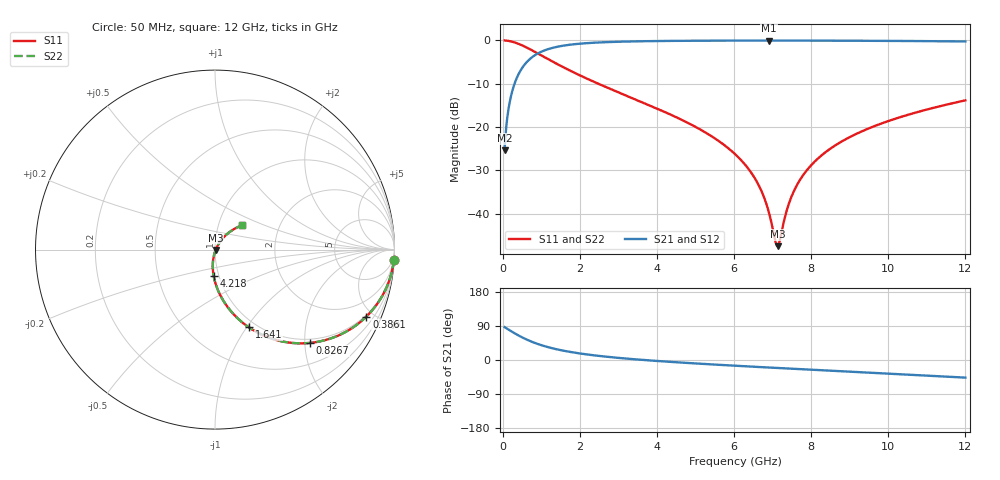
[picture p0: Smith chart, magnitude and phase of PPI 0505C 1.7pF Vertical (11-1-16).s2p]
# GHz S MA R 50
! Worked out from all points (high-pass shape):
!   1601 points, 50 MHz to 12 GHz, reference 50 ohm
!   highest |S21| = -0.04 dB at 6.906 GHz (marker M1); lowest = -25.3 dB at 50 MHz (marker M2)
!   |S21| within 3 dB of the highest: 907.1 MHz to end of sweep
!   lowest |S11| = -47.5 dB at 7.13 GHz (marker M3), VSWR 1.01, Z = 50.4 - j0.142 ohm
!   |S11| at or under -10 dB: 2.477 GHz to end of sweep
!   |S22| runs from -47.5 to 0.0 dB; largest |S21 - S12| = 0
!   S11 on the Smith chart (normalised r, x): 50 MHz: 1, -35; 386.1 MHz: 0.91, -4.55; 826.8 MHz: 0.91, -2.11; 1.641 GHz: 0.92, -1.02; 4.218 GHz: 0.94, -0.29; 12 GHz: 1.30, +0.37
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0.05  0.9985 -3.2  0.05403 86.7  0.05403 86.7  0.9985 -3.2
0.1919063  0.979 -12.3  0.2034 77.7  0.2034 77.7  0.979 -12.3
0.3860938  0.9221 -23.9  0.3862 66.1  0.3862 66.1  0.9221 -23.9
0.5802812  0.8451 -34.0  0.5336 55.9  0.5336 55.9  0.8451 -34.0
0.82675  0.7408 -44.6  0.6704 45.3  0.6704 45.3  0.7408 -44.6
1.207656  0.5974 -56.8  0.8001 33.1  0.8001 33.1  0.5974 -56.8
1.640844  0.4728 -66.4  0.879 23.3  0.879 23.3  0.4728 -66.4
2.044156  0.3866 -73.0  0.9198 16.6  0.9198 16.6  0.3866 -73.0
4.038312  0.1606 -91.7  0.9836 -2.8  0.9836 -2.8  0.1606 -91.7
4.217562  0.1482 -92.8  0.9855 -4.0  0.9855 -4.0  0.1482 -92.8
5.285594  0.08501 -98.4  0.9925 -10.8  0.9925 -10.8  0.08501 -98.4
6.025  0.04866 -100.6  0.9946 -15.1  0.9946 -15.1  0.04866 -100.6
6.56275  0.02456 -98.6  0.9953 -18.0  0.9953 -18.0  0.02456 -98.6
6.756938  0.0163 -94.6  0.9954 -19.1  0.9954 -19.1  0.0163 -94.6
6.906313  0.01024 -86.1  0.9954 -19.9  0.9954 -19.9  0.01024 -86.1
7.063156  0.004985 -53.7  0.9954 -20.7  0.9954 -20.7  0.004985 -53.7
7.130375  0.004205 -19.5  0.9953 -21.1  0.9953 -21.1  0.004205 -19.5
7.51875  0.01683 52.0  0.9951 -23.1  0.9951 -23.1  0.01683 52.0
8.019156  0.03696 57.3  0.9943 -25.7  0.9943 -25.7  0.03696 57.3
8.825781  0.06938 56.1  0.9922 -29.9  0.9922 -29.9  0.06938 56.1
10.01331  0.1176 51.4  0.9872 -36.0  0.9872 -36.0  0.1176 51.4
12  0.2031 41.8  0.9723 -46.5  0.9723 -46.5  0.2031 41.8
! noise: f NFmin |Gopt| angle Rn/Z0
0.05  0.0008959  0.954  1.726  0.004378
1.372  0.005506  0.7548  5.61  0.004526
2.701  0.008672  0.7016  9.165  0.005659
4.031  0.01147  0.67  12.78  0.006603
5.36  0.0141  0.6488  16.37  0.007474
6.682  0.01665  0.6344  19.88  0.008328
8.012  0.01922  0.6248  23.36  0.009211
9.341  0.02184  0.6193  26.76  0.01015
10.67  0.02456  0.6171  30.09  0.01118
12  0.02743  0.618  33.35  0.01234
